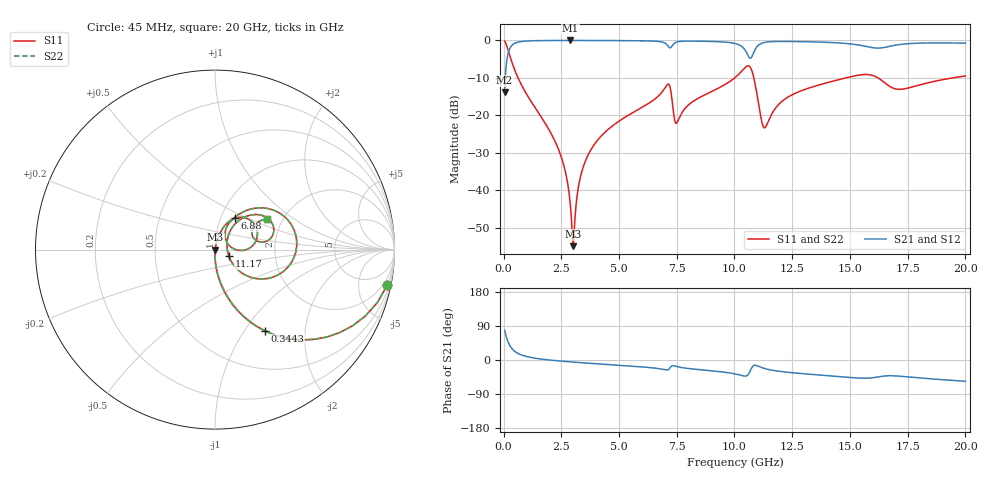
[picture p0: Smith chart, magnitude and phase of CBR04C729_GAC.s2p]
! S-parameter model data by Modelithics Inc.  support@modelithics.com 813-866-6335  Tampa FL USA
! S-Parameter data specifications:
! Substrate: 20-mil Rogers 4350B, substrate thickness, H=0.508mm, Dielectric constant, Er=3.75
! PCB Mounting Pad Footprint: Pad width, PadW=0.52mm , Pad length, PadL=0.52mm , Pad gap, PadG (edge-to-edge)=0.28mm , Reference planes=1.32mm apart
#  GHz  S  MA  R 50
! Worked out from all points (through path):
!   801 points, 45 MHz to 20 GHz, reference 50 ohm
!   highest |S21| = -0.02 dB at 2.889 GHz (marker M1); lowest = -13.9 dB at 45 MHz (marker M2)
!   group delay of S21, straight-line fit = 9.15 ps
!   lowest |S11| = -55.0 dB at 3.013 GHz (marker M3), VSWR 1.00, Z = 50.2 - j0.0201 ohm
!   |S11| at or under -10 dB: 626.4 MHz to 10.01 GHz (9.385 GHz wide, 176 % of centre); 10.84 GHz to 14.83 GHz (3.989 GHz wide, 31.1 % of centre); 16.21 GHz to 19.46 GHz (3.248 GHz wide, 18.2 % of centre)
!   |S22| runs from -55.0 to -0.2 dB; largest |S21 - S12| = 0
!   S11 on the Smith chart (normalised r, x): 45 MHz: 0.99, -9.63; 344.3 MHz: 0.99, -1.24; 6.88 GHz: 1.17, +0.43; 11.17 GHz: 1.16, -0.09; 20 GHz: 1.66, +0.64
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0.045  0.9794 -11.7  0.2021 78.3  0.2021 78.3  0.9794 -11.7
0.344325  0.53 -58.6  0.8474 31.4  0.8474 31.4  0.53 -58.6
0.8432  0.2322 -77.9  0.9717 11.9  0.9717 11.9  0.2322 -77.9
2.364769  0.03597 -89.8  0.9977 -2.3  0.9977 -2.3  0.03597 -89.8
2.689037  0.01694 -88.3  0.9981 -3.9  0.9981 -3.9  0.01694 -88.3
2.888587  0.006525 -79.4  0.9981 -4.9  0.9981 -4.9  0.006525 -79.4
3.013306  0.001787 -6.4  0.9981 -5.5  0.9981 -5.5  0.001787 -6.4
3.387462  0.01761 76.6  0.9978 -7.2  0.9978 -7.2  0.01761 76.6
4.310381  0.0561 76.6  0.996 -11.1  0.996 -11.1  0.0561 76.6
6.704981  0.1808 62.7  0.9687 -22.6  0.9687 -22.6  0.1808 62.7
6.879588  0.2075 57.5  0.9493 -24.4  0.9493 -24.4  0.2075 57.5
7.153969  0.2599 26.8  0.8175 -24.8  0.8175 -24.8  0.2599 26.8
7.503181  0.07926 37.7  0.9523 -17.4  0.9523 -17.4  0.07926 37.7
10.0225  0.3182 46.3  0.9096 -36.7  0.9096 -36.7  0.3182 46.3
10.4216  0.4218 27.2  0.7703 -42.2  0.7703 -42.2  0.4218 27.2
10.69598  0.4322 -9.4  0.5789 -26.9  0.5789 -26.9  0.4322 -9.4
11.16991  0.08574 -25.4  0.9143 -19.9  0.9143 -19.9  0.08574 -25.4
11.34452  0.0696 16.7  0.9453 -23.2  0.9453 -23.2  0.0696 16.7
13.36496  0.2387 48.3  0.9557 -38.1  0.9557 -38.1  0.2387 48.3
15.65979  0.3505 24.3  0.8355 -48.0  0.8355 -48.0  0.3505 24.3
16.68248  0.2475 10.3  0.8277 -41.7  0.8277 -41.7  0.2475 10.3
20  0.3354 30.3  0.9209 -56.1  0.9209 -56.1  0.3354 30.3
